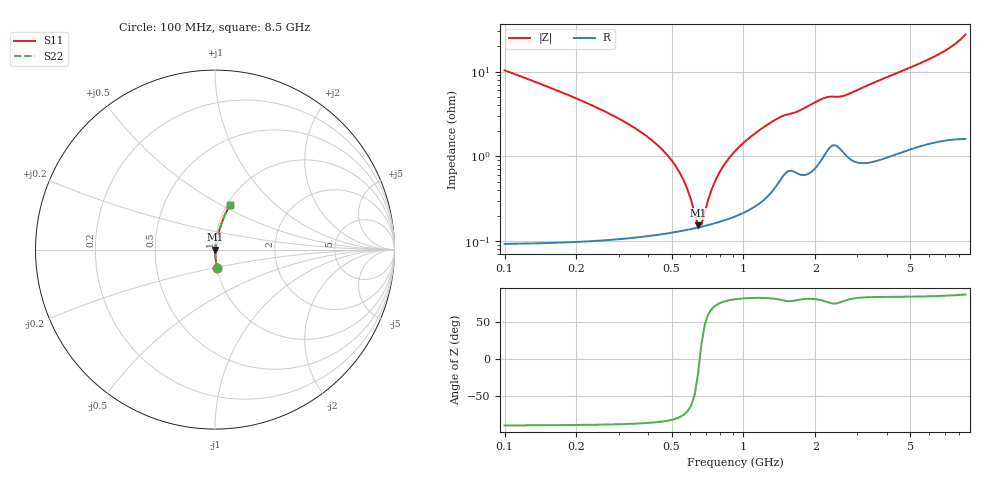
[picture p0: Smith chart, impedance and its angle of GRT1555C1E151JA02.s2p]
!Murata Part Number: GRT1555C1E151JA02
!These Parameters are Measured in Series Mode Connection
!Data Generated on Jun 19, 2026
!  o--ll--o
!Port1  Port2
!  o------o
!Operation Temp=25[degC], DC Bias Voltage=0[V]
!Freq. Start=100[MHz] Stop=9[GHz] 401[Steps]
# Hz S RI R 50
!Freq.(Hz) S11(Real) S11(Imag) S21(Real) S21(Imag) S12(Real) S12(Imag) S22(Real) S22(Imag)
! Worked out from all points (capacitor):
!   401 points, 100 MHz to 8.5 GHz, reference 50 ohm
!   read as one part in series: C = 150 pF near 142 MHz
!   lowest |Z| = 153 mohm at 646 MHz (marker M1)
!   series resonance near 656.3 MHz, so ESL is about 390 pH
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1e8  0.0115 -0.1023  0.9885 0.1023  0.9885 0.1023  0.0115 -0.1023
2.26e8  0.00269 -0.0412  0.9973 0.0412  0.9973 0.0412  0.00269 -0.0412
4.78e8  0.00133 -0.0104  0.9987 0.0104  0.9987 0.0104  0.00133 -0.0104
5.41e8  0.00134 -0.00627  0.9987 0.00627  0.9987 0.00627  0.00134 -0.00627
6.25e8  0.00141 -0.00157  0.9986 0.00157  0.9986 0.00157  0.00141 -0.00157
6.46e8  0.00144 -0.000506  0.9986 0.000506  0.9986 0.000506  0.00144 -0.000506
6.67e8  0.00147 0.000528  0.9985 -0.000528  0.9985 -0.000528  0.00147 0.000528
6.88e8  0.00151 0.00153  0.9985 -0.00153  0.9985 -0.00153  0.00151 0.00153
7.51e8  0.00162 0.00439  0.9984 -0.00439  0.9984 -0.00439  0.00162 0.00439
8.14e8  0.00177 0.00705  0.9982 -0.00705  0.9982 -0.00705  0.00177 0.00705
9.4e8  0.00213 0.012  0.9979 -0.012  0.9979 -0.012  0.00213 0.012
1.045e9  0.00253 0.0158  0.9975 -0.0158  0.9975 -0.0158  0.00253 0.0158
1.192e9  0.00333 0.0209  0.9967 -0.0209  0.9967 -0.0209  0.00333 0.0209
1.36e9  0.005 0.0265  0.995 -0.0265  0.995 -0.0265  0.005 0.0265
1.507e9  0.00724 0.0298  0.9928 -0.0298  0.9928 -0.0298  0.00724 0.0298
2.179e9  0.0123 0.0466  0.9877 -0.0466  0.9877 -0.0466  0.0123 0.0466
2.578e9  0.0139 0.0485  0.9861 -0.0485  0.9861 -0.0485  0.0139 0.0485
2.914e9  0.0118 0.0566  0.9882 -0.0566  0.9882 -0.0566  0.0118 0.0566
4.3e9  0.0187 0.0906  0.9813 -0.0906  0.9813 -0.0906  0.0187 0.0906
5.707e9  0.0296 0.1255  0.9704 -0.1255  0.9704 -0.1255  0.0296 0.1255
7.114e9  0.0457 0.1707  0.9543 -0.1707  0.9543 -0.1707  0.0457 0.1707
8.5e9  0.0825 0.2475  0.9175 -0.2475  0.9175 -0.2475  0.0825 0.2475
